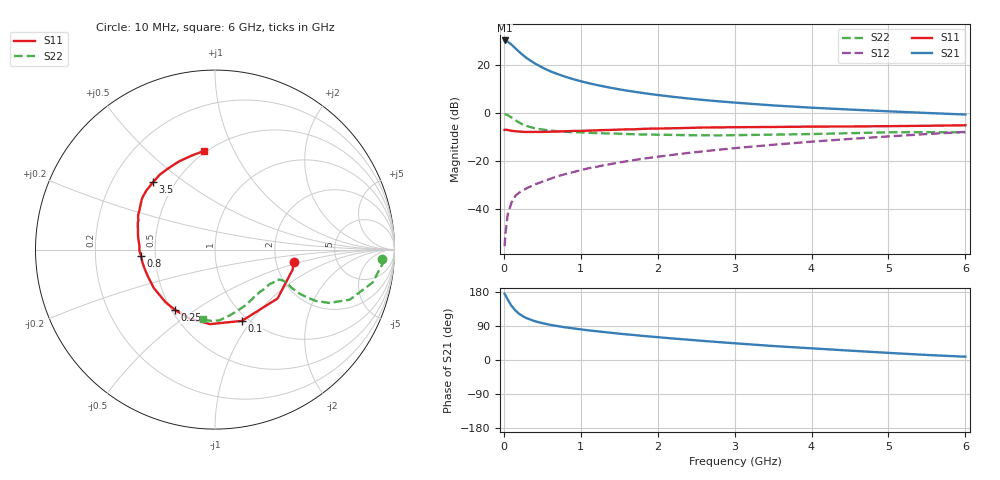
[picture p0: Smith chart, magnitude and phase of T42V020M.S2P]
! Infineon Technologies  Discrete & RF Semiconductors
! BFR182T
! Si NPN RF Bipolar Junction Transistor in SC75
! VCE = 2 V  IC = 20 mA
! Common Emitter S-Parameters:  October  1999
# GHz  S  MA  R  50
!  f  S11  S21  S12  S22
! GHz  MAG  ANG  MAG  ANG  MAG  ANG  MAG  ANG
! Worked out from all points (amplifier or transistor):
!   36 points, 10 MHz to 6 GHz, reference 50 ohm
!   highest |S21| = 30.1 dB at 10 MHz (marker M1)
!   |S21| within 3 dB of that: start of sweep to 141.2 MHz
!   unconditionally stable (mu >= 1): start of sweep to 10.45 MHz; 488.1 MHz to 3.931 GHz
!   at 250 MHz: K = 0.73, MSG = 28.1 dB, |S12| = -32.2 dB
!   at 1.4 GHz: K = 1.19, MAG = 13.2 dB, |S12| = -21.2 dB
!   at 6 GHz: K = 0.87, MSG = 3.6 dB, |S12| = -7.9 dB
!   S11 on the Smith chart (normalised r, x): 10 MHz: 2.51, -0.44; 100 MHz: 0.93, -0.90; 250 MHz: 0.52, -0.42; 800 MHz: 0.41, -0.03; 3.5 GHz: 0.38, +0.38; 6 GHz: 0.49, +0.77
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0.01  0.4438 -9.1  32.01 174.8  0.0017 79.2  0.9308 -3.1
0.02  0.4467 -14.4  31.68 171.7  0.003 90.4  0.9365 -4.9
0.05  0.4424 -38.0  30.37 159.5  0.0077 81.4  0.8971 -11.8
0.1  0.4244 -69.3  26.19 143.0  0.0137 69.3  0.801 -20.4
0.15  0.4162 -93.8  21.98 130.6  0.0189 64.9  0.7029 -25.0
0.2  0.4096 -110.3  18.52 121.8  0.0221 62.4  0.6292 -27.0
0.25  0.4032 -123.4  15.78 115.3  0.0245 60.6  0.5717 -27.5
0.3  0.4025 -133.3  13.67 110.1  0.0274 62.2  0.5333 -27.5
0.4  0.4025 -147.9  10.73 102.5  0.0324 62.8  0.4795 -26.6
0.5  0.4023 -157.2  8.766 97.3  0.0372 65.0  0.4516 -25.4
0.6  0.4061 -164.5  7.379 92.9  0.0425 65.7  0.4311 -24.8
0.7  0.4108 -170.1  6.396 89.4  0.0484 68.0  0.4166 -24.5
0.8  0.4144 -175.3  5.636 86.2  0.0534 68.8  0.4059 -24.7
0.9  0.4217 -179.5  5.028 83.5  0.0586 70.1  0.3968 -24.9
1.1  0.4286 173.3  4.156 78.2  0.0706 70.7  0.3866 -26.1
1.3  0.4395 167.7  3.546 73.8  0.082 71.3  0.3759 -27.9
1.6  0.4559 160.6  2.905 67.6  0.099 71.5  0.3642 -31.2
2.2  0.4791 150.8  2.157 56.7  0.1348 71.0  0.3489 -40.0
3.5  0.5097 132.7  1.43 36.9  0.2177 66.4  0.3536 -61.5
4.5  0.522 119.9  1.173 24.7  0.2879 60.6  0.3786 -78.7
5.5  0.5397 104.0  0.997 13.3  0.3635 53.8  0.3979 -93.3
6  0.5531 96.3  0.925 8.7  0.4028 49.6  0.3943 -99.6
